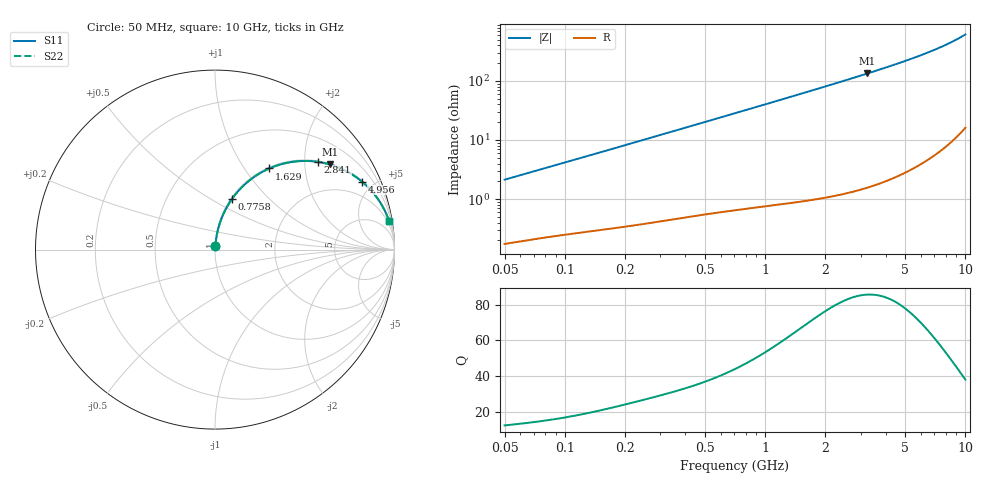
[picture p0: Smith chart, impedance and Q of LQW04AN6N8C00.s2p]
!Murata Part Number: LQW04AN6N8C00
!These Parameters are Measured in Series Mode Connection
!  o--[Z]--o
!Port1  Port2
!  o-------o
!Freq. Start=50[MHz] Stop=10[GHz], 401[Steps]
# Hz S RI R 50
!Freq.(Hz)	S 11(Real)	S 11(Imag)	S 21(Real)	S 21(Imag)	S 12(Real)	S 12(Imag)	S 22(Real)	S 22(Imag)
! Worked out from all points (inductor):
!   401 points, 50 MHz to 10 GHz, reference 50 ohm
!   read as one part in series: L = 6.7 nH near 51.34 MHz
!   highest Q = 85.7 at 3.244 GHz (marker M1), where L = 6.56 nH
!   S11 on the Smith chart (normalised r, x): 50 MHz: 1.00, +0.04; 775.8 MHz: 1.01, +0.62; 1.629 GHz: 1.02, +1.31; 2.841 GHz: 1.03, +2.32; 4.956 GHz: 1.05, +4.30; 10 GHz: 1, +12
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5e7  0.00219 0.0211  0.9978 -0.0211  0.9978 -0.0211  0.00219 0.0211
1.214486e8  0.0052 0.0497  0.9948 -0.0497  0.9948 -0.0497  0.0052 0.0497
1.956524e8  0.00965 0.0789  0.9904 -0.0789  0.9904 -0.0789  0.00965 0.0789
2.949953e8  0.0181 0.1171  0.9819 -0.1171  0.9819 -0.1171  0.0181 0.1171
4.628099e8  0.0384 0.1785  0.9616 -0.1785  0.9616 -0.1785  0.0384 0.1785
7.071068e8  0.0796 0.2594  0.9204 -0.2594  0.9204 -0.2594  0.0796 0.2594
7.758058e8  0.0932 0.2802  0.9068 -0.2802  0.9068 -0.2802  0.0932 0.2802
9.463279e8  0.1304 0.3272  0.8696 -0.3272  0.8696 -0.3272  0.1304 0.3272
1.139142e9  0.1766 0.3727  0.8234 -0.3727  0.8234 -0.3727  0.1766 0.3727
1.353197e9  0.2309 0.4136  0.7691 -0.4136  0.7691 -0.4136  0.2309 0.4136
1.628911e9  0.3023 0.4521  0.6977 -0.4521  0.6977 -0.4521  0.3023 0.4521
1.717543e9  0.3251 0.4615  0.6749 -0.4615  0.6749 -0.4615  0.3251 0.4615
1.9608e9  0.3859 0.4803  0.6141 -0.4803  0.6141 -0.4803  0.3859 0.4803
2.23851e9  0.4511 0.4914  0.5489 -0.4914  0.5489 -0.4914  0.4511 0.4914
2.841223e9  0.5734 0.4887  0.4266 -0.4887  0.4266 -0.4887  0.5734 0.4887
3.243629e9  0.6398 0.4743  0.3602 -0.4743  0.3602 -0.4743  0.6398 0.4743
4.171863e9  0.7541 0.4246  0.2459 -0.4246  0.2459 -0.4246  0.7541 0.4246
4.955797e9  0.8194 0.3784  0.1806 -0.3784  0.1806 -0.3784  0.8194 0.3784
6.045081e9  0.8799 0.318  0.1201 -0.318  0.1201 -0.318  0.8799 0.318
7.276762e9  0.9226 0.2588  0.0774 -0.2588  0.0774 -0.2588  0.9226 0.2588
8.418147e9  0.948 0.2122  0.052 -0.2122  0.052 -0.2122  0.948 0.2122
1e10  0.97 0.1579  0.03 -0.1579  0.03 -0.1579  0.97 0.1579
